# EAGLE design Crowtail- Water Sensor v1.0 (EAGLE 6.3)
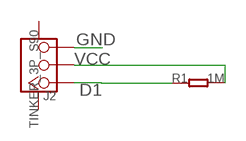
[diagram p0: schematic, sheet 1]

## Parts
J2  TINKER_3P_S90  [TINKER_3P_S90]
R1  1M  R0603  [0603]

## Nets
D1: J2.1 R1.1
GND: J2.3
VCC: J2.2 R1.2
Unconnected: J2.SS1 J2.SS2

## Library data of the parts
J2 = Connector:TINKER_3P_S90
R1 = CPT_SMD:R0603

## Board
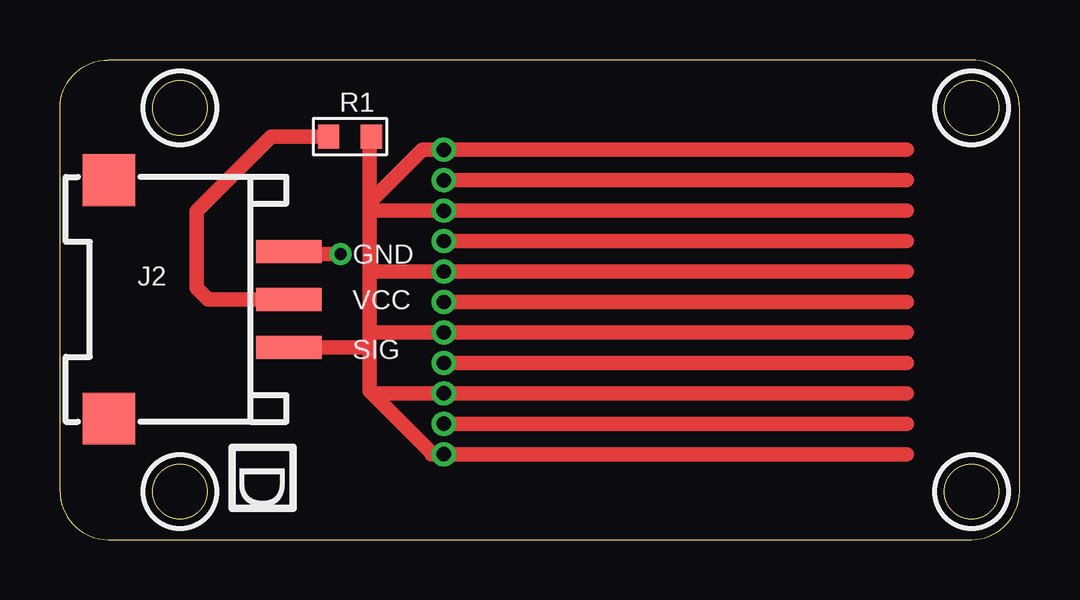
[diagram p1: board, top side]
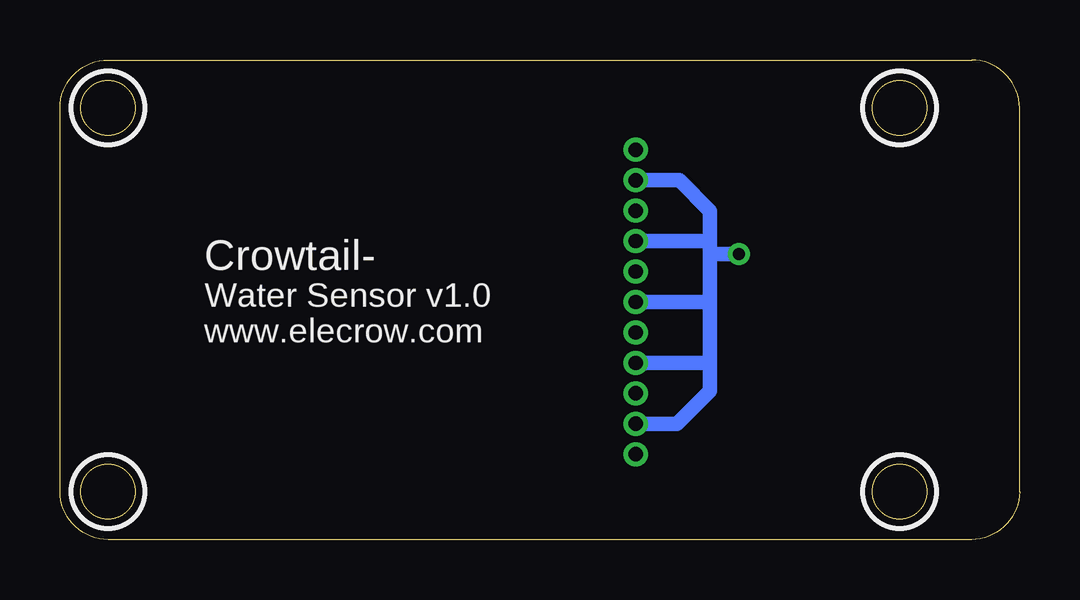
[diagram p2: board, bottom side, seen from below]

Size 40 x 20 mm. Coordinates in mm from the lower left corner, seen from the top.
Outline: 0,2 0,18 arc-90 2,20 38,20 arc-90 40,18 40,2 arc-90 38,0 2,0 arc-90 0,2
Outline: circle at 5,18 radius 1.14
Outline: circle at 5,2 radius 1.14
Outline: circle at 38,18 radius 1.14
Outline: circle at 38,2 radius 1.14
Copper layers (1*16): Top 0.035mm / dielectric 1.5mm / Bottom 0.035mm
Design rules "default *": minimum track width 10mil, minimum drill 16mil, track to track 8mil, track to pad 8mil, pad to pad 8mil, via to via 8mil, smd to smd 8mil, copper to edge 20mil, drill to drill 8mil, minimum pad ring 10mil, minimum via ring 8mil, stop-mask expansion 2mil, vias tented up to drill 100mil, thermal gap 10mil
tRestrict: area 3.5,16.5 to 6.5,19.5; area 3.5,0.5 to 6.5,3.5; area 36.5,16.5 to 39.5,19.5; area 36.5,0.5 to 39.5,3.5
bRestrict: area 3.5,16.5 to 6.5,19.5; area 3.5,0.5 to 6.5,3.5; area 36.5,16.5 to 39.5,19.5; area 36.5,0.5 to 39.5,3.5

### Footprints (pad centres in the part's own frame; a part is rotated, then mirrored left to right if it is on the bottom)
TINKER_3P_S90 = smd 0.965 x 2.74: 1 -1.984,-4.545; 2 0.016,-4.545; 3 2.016,-4.545 | smd 2.159 x 2.184: SS1 -4.958,2.955; SS2 4.99,2.955
0603 = smd 0.889 x 1.016: 1 -0.889,0; 2 0.889,0

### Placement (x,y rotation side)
J2  5,10 90 top
R1  12.09,16.8 180 top

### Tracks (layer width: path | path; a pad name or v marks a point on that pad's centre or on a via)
D1  (via drill 0.6)
  Top 0.61: 35.31,11.18 v16,11.18 13.13,11.18 12.9,11.4 | 35.31,13.72 v16,13.72 13.02,13.72 | v16,8.64 35.31,8.64 | 35.31,3.56 v16,3.56 15.49,3.56 15.49,3.61 13.15,5.95 | 35.31,16.26 v16,16.26 15.11,16.26 12.95,14.1 13.02,14.04 13.02,13.72 | 35.31,6.1 v16,6.1 13.3,6.1 13.15,5.95 | 15.49,8.64 v16,8.64 | 13.15,5.95 12.9,6.2 12.9,8.1 | 12.95,16.78 R1.1 12.9,16.73 12.9,13.6 | 12.9,8.1 12.9,8.6 | 12.9,8.6 12.9,11.4 | 12.9,11.4 12.9,13.6 | 13.02,13.72 12.9,13.6 | v16,8.64 12.94,8.64 12.9,8.6 | J2.1 12.82,8.02 12.9,8.1
GND  (via drill 0.51, 0.6)
  Top 0.61: v16,4.83 35.31,4.83 | 35.31,12.45 v16,12.45 | v16,9.91 35.31,9.91 | v16,7.37 35.31,7.37 | v16,14.99 35.31,14.99 | v11.7,11.9 9.66,11.9 J2.3
  Bottom 0.61: v16,4.83 14.27,4.83 12.9,6.2 12.9,7.3 | v16,12.45 15.06,12.45 | v16,12.45 15.16,12.45 | v16,9.91 12.99,9.91 12.9,10 | v16,12.45 12.95,12.45 12.9,12.5 | v16,7.37 12.97,7.37 12.9,7.3 | 12.9,7.3 12.9,10 | 12.9,10 12.9,11.9 12.8,11.9 | 12.8,11.9 11.9,11.9 v11.7,11.9 | v16,14.99 14.19,14.99 12.9,13.7 12.9,12.5 | 12.9,12.5 12.9,12 12.8,11.9
VCC
  Top 0.61: J2.2 6.18,10.02 5.7,10.5 5.7,13.7 8.8,16.8 R1.2

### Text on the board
tPlace: GND | VCC | SIG | D
bPlace: Crowtail- | Water Sensor v1.0 | www.elecrow.com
